PROGRAM MAIN
VAR
	ENABLE:BOOL;

//RECIPE
PROCESS:PROCESS;
PROCESS_EN:BOOL;
PROCESS_RUN:BOOL;
PROCESS_STOP:BOOL;

P_NO:INT;

CYCLE_EN:BOOL;
CYCLE_NUM:INT;
CYCLE_START_STEP_NO:INT;

STEP_NO:INT;
NEXTSTEP_EN:BOOL;

UPS:FB_S_UPS_BAPI;

END_VAR

//UPS
UPS(
	sNetID:= , 
	iPLCPort:= 851, 
	tTimeout:= , 
	eUpsMode:= eSUPS_WrPersistData_shutdown, 
	ePersistentMode:= , 
	tRecoverTime:= T#10S, 
	bPowerFailDetect=> , 
	eState=> , 
	nCapacity=> , 
	bBusy=> , 
	bError=> , 
	nErrID=> );

//******************************IO*********************************
	IO_EXCHANGE();

//*****************************CONFIGURATION***********************
	IL();

//*****************************INTERLOCK***************************
	Temp();
	
//*****************************PROCESS*****************************
	PROCESS_RUN:=GV.Process_Start AND NOT GV.ALARM_OCC AND GV.NDI.GV1_CLOSE;
	PROCESS_STOP:=GV.Process_Stop OR GV.ALARM_OCC;

	//PROCESS ENABLE
	IF PROCESS_RUN AND NOT PROCESS_EN
		THEN
		CYCLE_NUM := 0;
		STEP_NO:=1;
		P_NO:=1;
		PM.ProcessFeedBack.ProcessFinished:=FALSE;
	END_IF
		IF PROCESS_RUN AND NOT PROCESS_EN
		THEN
		PROCESS_EN:=TRUE;		
	END_IF;
	
	IF PROCESS_STOP
		THEN
		CYCLE_NUM:=0;
		CYCLE_EN:=FALSE;
		PROCESS_EN:=FALSE;
		PROCESS_RUN:=FALSE;
	END_IF;
	IF NOT PM.ProcessFeedBack.ProcessFinished
		THEN 
			PM.ProcessFeedBack.CurrentStepNo:=STEP_NO;
		ELSE
			PM.ProcessFeedBack.CurrentStepNo:=STEP_NO-1;
	END_IF
	
	IF PROCESS_EN
		THEN 
		PM.ProcessFeedBack.ProcessStart:=TRUE;
		PM.ProcessFeedBack.CurrentStepstart:=TRUE;
		ELSE
			PM.ProcessFeedBack.ProcessStart:=FALSE;
			PM.ProcessFeedBack.CurrentStepstart:=FALSE;
		END_IF
	
	IF GV.Step_Num<STEP_NO 
		THEN 	
		PM.ProcessFeedBack.ProcessFinished:=TRUE;
	END_IF
	IF  GV.ALARM_OCC
		THEN
		PROCESS_EN:=FALSE;	
		
	END_IF
	
	IF STEP_NO<1 OR STEP_NO >100
		THEN 
		STEP_NO:=1;
	END_IF
	
	//CYCLE初始化
	IF GV.SetpArray[STEP_NO].CycleStart AND CYCLE_EN=FALSE
		THEN 
		CYCLE_EN				:=	TRUE;
		CYCLE_START_STEP_NO		:=	STEP_NO;
		CYCLE_NUM				:=	GV.SetpArray[STEP_NO].CycleNumber;
	END_IF;	
	
	//STEP
	PROCESS(
	ENABLE			:= 	PROCESS_EN, 
	NEXTSTEP_EN		:=	NEXTSTEP_EN,
	Alarm_RST		:=	UI.Warning_And_Alarm_RST,
	PMStableTime	:=	UI.PMConfig.PMStableTime,
	STEP_DATA		:= 	GV.SetpArray[STEP_NO],  
	);
	
	//PROCESS FLOW	
	CASE P_NO OF
		1:	IF NOT PROCESS_EN 
				THEN 
				P_NO:=100;
				ELSE
				P_NO:=2;	
			END_IF;
			NEXTSTEP_EN:=FALSE;
			
		2:	IF PROCESS.NEXTSTEP 
				THEN 
				PM.ProcessFeedBack.CurrentStepFinished:=TRUE;
				PM.ProcessFeedBack.CurrentStepstart:=FALSE;
				P_NO:=3;
			END_IF;
			
		3:	IF CYCLE_EN
			THEN
				P_NO:=10;
				ELSE
				P_NO:=20;
			END_IF
		
		10:	IF GV.SetpArray[STEP_NO].CycleEnd 
				THEN 
				P_NO:=11; 
				ELSE
				P_NO:=20; 
			END_IF;	
		
		11:	IF CYCLE_NUM=0 
				THEN 
				P_NO:=20; 
				CYCLE_EN:=FALSE;
				ELSE
				CYCLE_NUM:=CYCLE_NUM-1; 
				P_NO:=21; 
			END_IF;	
				
		20:	STEP_NO:=STEP_NO+1;
			NEXTSTEP_EN:=TRUE;
			P_NO:=1; 
			PM.ProcessFeedBack.CurrentStepstart:=TRUE;
			PM.ProcessFeedBack.CurrentStepFinished:=FALSE;
			
		21:	STEP_NO:=CYCLE_START_STEP_NO;
			NEXTSTEP_EN:=TRUE;
			P_NO:=1;
		
		100:;	
	END_CASE;	
		
	
	IF	PROCESS_EN
		THEN
//******************工艺参数赋值***************
		//APC
		GV.	AO.	APC.TARGET_PRESSURE	:=	PROCESS.APC_PRESSURE;
		GV.	AO.	APC.TARGET_POSITION	:=	PROCESS.APC_POSITION;
		IF GV_IL.APC_EN THEN 
		GV.AO.	APC.	Control_Mode	:=	PROCESS.APC_CONTROL_MODE	;
		ELSE 
		GV.AO.	APC.	Control_Mode	:=	3	;
		END_IF
		
		//MFC
		GV.AO.MFC1_Flow_Setpoint	:=	PROCESS.MFC1_SV;
(*		GV.AO.MFC2_Flow_Setpoint	:=	PROCESS.MFC2_SV;
		GV.AO.MFC3_Flow_Setpoint	:=	PROCESS.MFC3_SV;
//		GV.AO.MFC4_Flow_Setpoint	:=	PROCESS.MFC4_SV;
		GV.AO.MFC5_Flow_Setpoint	:=	PROCESS.MFC5_SV;
		GV.AO.MFC6_Flow_Setpoint	:=	PROCESS.MFC6_SV;
		GV.AO.MFC7_Flow_Setpoint	:=	PROCESS.MFC7_SV;
	//	GV.AO.MFC8_Flow_Setpoint	:=	PROCESS.MFC8_SV;
	//	GV.AO.MFC9_Flow_Setpoint	:=	PROCESS.MFC9_SV;
*)		
//LID HEATER
		GV.AO.LID_Temp_SV			:=	PROCESS.LID_TEMP;		
		
//CHAMBER HEATER
		GV.AO.	Chamber_Temp1_SV	:=	
		GV.AO.	Chamber_Temp2_SV	:=	
		GV.AO.	Chamber_Temp3_SV	:=	PROCESS.WALL_TEMP;
//STAGE
		GV.AO.Stage_Temp1_SV	 	:=	PROCESS.STAGE_TEMP1;
		GV.AO.Stage_Temp1_SV	 	:=	PROCESS.STAGE_TEMP2;	
		GV.AO.Stage_Temp1_SV	 	:=	PROCESS.STAGE_TEMP3;	
		GV.AO.Stage_Temp1_SV	 	:=	PROCESS.STAGE_TEMP4;		
		
//************************TOLERANCE 赋值****************
		

//************************VALVE动作****************
		GV.NDO.AV1	:=	FALSE	;//	(	GV.AO.MFC1_Flow_Setpoint>0	)	AND	PM.INFO.Alarm.TOLERANCE_MFC1	AND	GV_IL.AV1_EN	;
		GV.NDO.AV2	:=			(	GV.AO.MFC1_Flow_Setpoint>0	)	AND	NOT PM.INFO.Alarm.TOLERANCE_MFC1	AND	GV_IL.AV2_EN	;
		GV.NDO.AV3	:=	FALSE	;//(	GV.AO.MFC1_Flow_Setpoint>0	)	AND	PM.INFO.Alarm.TOLERANCE_MFC1	AND	GV_IL.AV3_EN	;
		GV.NDO.AV4	:=	FALSE	;//	(	GV.AO.MFC2_Flow_Setpoint>0	)	AND	PM.INFO.Alarm.TOLERANCE_MFC2	AND	GV_IL.AV4_EN	;
		GV.NDO.AV5	:=			(	GV.AO.MFC1_Flow_Setpoint>0	)	AND	NOT PM.INFO.Alarm.TOLERANCE_MFC1	AND	GV_IL.AV5_EN	;
		GV.NDO.AV26	:=			(	GV.AO.MFC1_Flow_Setpoint>0	)	AND	NOT PM.INFO.Alarm.TOLERANCE_MFC1	AND	GV_IL.AV26_EN	;

	END_IF

//TOL ALRM&WARNING
	PM.INFO.Alarm.TOLERANCE_PRESSURE			:=  PROCESS.PRESSURE_ALARM;
	PM.INFO.Alarm.TOLERANCE_MFC1				:=  PROCESS.MFC1_Alarm;
	PM.INFO.Alarm.TOLERANCE_WALL_TEMP			:=  PROCESS.WALL_TEMP_Alarm;
	PM.INFO.Alarm.TOLERANCE_LID_TEMP			:=  PROCESS.LID_TEMP_Alarm;
	PM.INFO.Alarm.TOLERANCE_STAGE_TEMP1			:=  PROCESS.STAGE_TEMP1_Alarm;
	PM.INFO.Alarm.TOLERANCE_STAGE_TEMP2			:=  PROCESS.STAGE_TEMP2_Alarm;
	PM.INFO.Alarm.TOLERANCE_STAGE_TEMP3			:=  PROCESS.STAGE_TEMP3_Alarm;
	PM.INFO.Alarm.TOLERANCE_STAGE_TEMP4			:=  PROCESS.STAGE_TEMP4_Alarm;
	
	PM.INFO.Warning.TOLERANCE_PRESSURE			:=  PROCESS.PRESSURE_WARNING;	
	PM.INFO.Warning.TOLERANCE_MFC1				:=  PROCESS.MFC1_WARNING;
	PM.INFO.Warning.TOLERANCE_WALL_TEMP			:=  PROCESS.WALL_TEMP_WARNING;	
	PM.INFO.Warning.TOLERANCE_LID_TEMP			:=  PROCESS.LID_TEMP_WARNING;	
	PM.INFO.Warning.TOLERANCE_STAGE_TEMP1		:=  PROCESS.STAGE_TEMP1_WARNING;		
	PM.INFO.Warning.TOLERANCE_STAGE_TEMP2		:=  PROCESS.STAGE_TEMP2_WARNING;	
	PM.INFO.Warning.TOLERANCE_STAGE_TEMP3		:=  PROCESS.STAGE_TEMP3_WARNING;		
	PM.INFO.Warning.TOLERANCE_STAGE_TEMP4		:=  PROCESS.STAGE_TEMP4_WARNING;

END_PROGRAM
